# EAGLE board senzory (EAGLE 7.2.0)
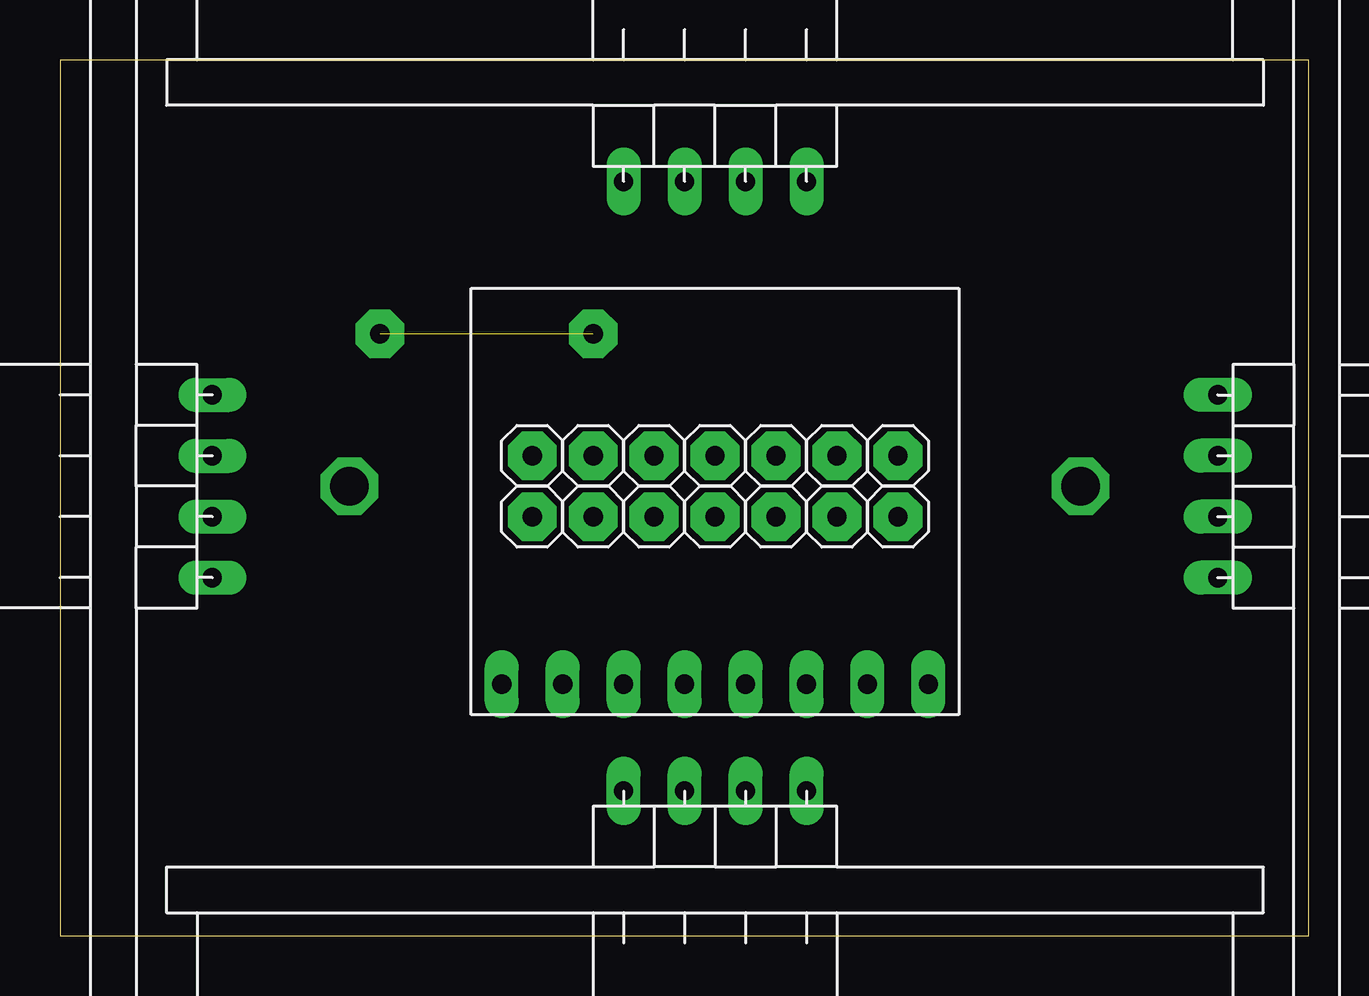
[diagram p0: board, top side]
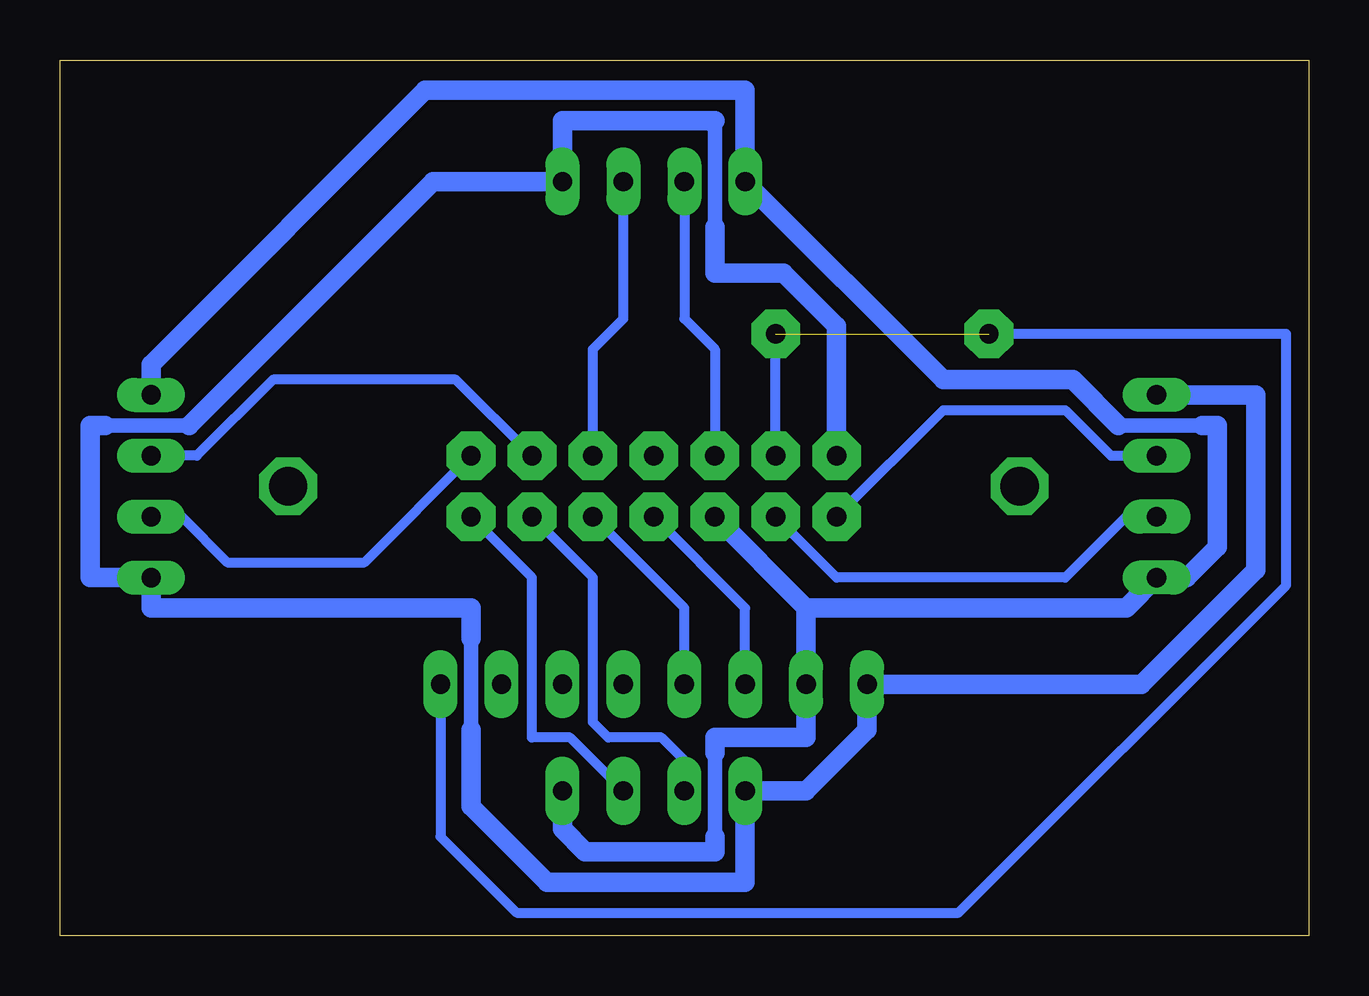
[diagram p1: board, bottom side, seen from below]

Size 52.06 x 36.5 mm. Coordinates in mm from the lower left corner, seen from the top.
Outline: 0,0 52.06,0 52.06,36.5 0,36.5 0,0
Copper layers (1*16): Top 0.035mm / dielectric 1.5mm / Bottom 0.035mm
Design rules "default": minimum track width 10mil, minimum drill 24mil, track to track 8mil, track to pad 8mil, pad to pad 8mil, via to via 8mil, smd to smd 8mil, copper to edge 40mil, drill to drill 8mil, minimum pad ring 10mil, minimum via ring 8mil, stop-mask expansion 4mil, vias tented up to drill 0mil, thermal gap 10mil

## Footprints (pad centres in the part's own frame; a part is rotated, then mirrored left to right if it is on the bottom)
WIFI = drill 0.8 pad 1.422 long: P$1 0,0; P$2 2.54,0; P$3 5.08,0; P$4 7.62,0; P$5 10.16,0; P$6 12.7,0; P$7 15.24,0; P$8 17.78,0
CON_4 = drill 0.8 pad 1.422 long: P$1 -8.89,5.08; P$2 -6.35,5.08; P$3 -3.81,5.08; P$4 -1.27,5.08
CON_1 = drill 0.8 pad 2.032 octagon: P$1 0,0

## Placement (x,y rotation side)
U$1  WIFI  [WIFI]  18.41,10.48 0 top
U$2  HC_SR  [CON_4]  22.23,36.51 180 top
U$3  HC_SR  [CON_4]  53.34,23.81 90 top
U$4  HC_SR  [CON_4]  1.27,13.65 270 top
U$5  HC_SR  [CON_4]  32.38,0.95 0 top
U$25  SDA  [CON_1]  29.84,17.46 270 top
U$26  INT  [CON_1]  22.23,20 270 top
U$27  5V  [CON_1]  19.68,20 270 top
U$28  GND  [CON_1]  24.77,17.46 270 top
U$29  ECHO  [CON_1]  24.77,20 270 top
U$30  TRIG  [CON_1]  29.84,20 270 top
U$31  ECHO  [CON_1]  32.38,20 270 top
U$32  TRIG  [CON_1]  34.92,20 270 top
U$33  SCL  [CON_1]  27.3,17.46 270 top
U$34  ECHO  [CON_1]  22.23,17.46 270 top
U$35  TRIG  [CON_1]  19.68,17.46 270 top
U$36  ECHO  [CON_1]  34.92,17.46 270 top
U$37  TRIG  [CON_1]  32.38,17.46 270 top
U$38  nic  [CON_1]  27.3,20 270 top

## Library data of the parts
U$1-U$5 U$25-U$38 = arduino

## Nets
N$1: U$1.P$1 U$2.P$1 U$3.P$1 U$4.P$1 U$5.P$1 U$27.P$1
N$2: U$1.P$2 U$2.P$4 U$3.P$4 U$4.P$4 U$5.P$4 U$28.P$1
N$3: U$2.P$2 U$30.P$1
N$4: U$2.P$3 U$29.P$1
N$5: U$3.P$2 U$32.P$1
N$6: U$3.P$3 U$31.P$1
N$7: U$4.P$2 U$35.P$1
N$8: U$4.P$3 U$34.P$1
N$9: U$5.P$2 U$37.P$1
N$10: U$5.P$3 U$36.P$1
N$11: U$1.P$3 U$33.P$1
N$12: U$1.P$4 U$25.P$1
N$13: U$1.P$8 U$26.P$1

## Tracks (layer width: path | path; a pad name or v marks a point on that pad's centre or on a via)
N$1
  Bottom 0.61: 34.92,8.57 34.92,12.38 | 50.16,21.27 46.67,21.27 | 24.77,29.53 24.77,33.66 25.08,33.97
  Bottom 0.813: U$27.P$1 19.68,25.4 21.91,27.62 24.77,27.62 24.77,29.53 | 24.77,33.97 25.08,33.97 31.11,33.97 U$2.P$1 36.51,31.43 46.67,21.27 | U$4.P$1 2.22,22.54 2.22,15.24 6.99,10.48 U$1.P$1 18.41,8.57 20.95,6.03 U$5.P$1 23.5,2.22 31.75,2.22 34.92,5.4 34.92,8.57 | 34.92,12.38 34.92,13.65 48.26,13.65 U$3.P$1 50.8,14.92 50.8,21.27 50.16,21.27
N$2
  Bottom 0.61: 24.77,7.62 24.77,4.13 | 4.45,21.27 7.94,21.27
  Bottom 0.813: U$3.P$4 48.26,23.81 36.83,35.24 23.5,35.24 U$2.P$4 15.24,23.18 9.84,23.18 7.94,21.27 | 20.95,13.65 U$1.P$2 20.95,8.26 24.77,8.26 24.77,7.62 | U$28.P$1 20.95,13.65 | 20.95,13.65 7.62,13.65 U$4.P$4 5.08,14.92 3.81,16.19 3.81,21.27 4.45,21.27 | U$5.P$4 31.11,4.45 30.16,3.49 24.77,3.49 24.77,4.13
N$3
  Bottom 0.406: U$30.P$1 29.84,24.45 28.57,25.72 U$2.P$2
N$4
  Bottom 0.406: U$2.P$3 26.04,25.72 24.77,24.45 U$29.P$1
N$5
  Bottom 0.406: U$32.P$1 39.37,15.56 45.09,15.56 46.99,17.46 U$3.P$2
N$6
  Bottom 0.406: U$31.P$1 35.56,23.18 43.18,23.18 46.35,20 U$3.P$3
N$7
  Bottom 0.406: U$35.P$1 15.24,21.91 10.16,21.91 8.26,20 U$4.P$2
N$8
  Bottom 0.406: U$4.P$3 7.62,17.46 10.16,14.92 19.68,14.92 U$34.P$1
N$9
  Bottom 0.406: U$37.P$1 29.84,14.92 29.84,8.89 29.21,8.26 26.99,8.26 26.04,7.3 U$5.P$2
N$10
  Bottom 0.406: U$36.P$1 32.38,14.92 32.38,8.26 30.8,8.26 U$5.P$3
N$11
  Bottom 0.406: U$1.P$3 23.5,13.65 U$33.P$1
N$12
  Bottom 0.406: U$1.P$4 26.04,13.65 U$25.P$1
N$13  (via drill 0.8 pad 2.03)  (1 unrouted)
  Bottom 0.406: U$1.P$8 36.2,4.13 33.02,0.95 14.61,0.95 0.95,14.61 0.95,25.08 v13.34,25.08 | U$26.P$1 v22.23,25.08
N$14  (via drill 1.6 pad 2.03)
  other vias: 42.55,18.73
N$15  (via drill 1.6 pad 2.03)
  other vias: 12.06,18.73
